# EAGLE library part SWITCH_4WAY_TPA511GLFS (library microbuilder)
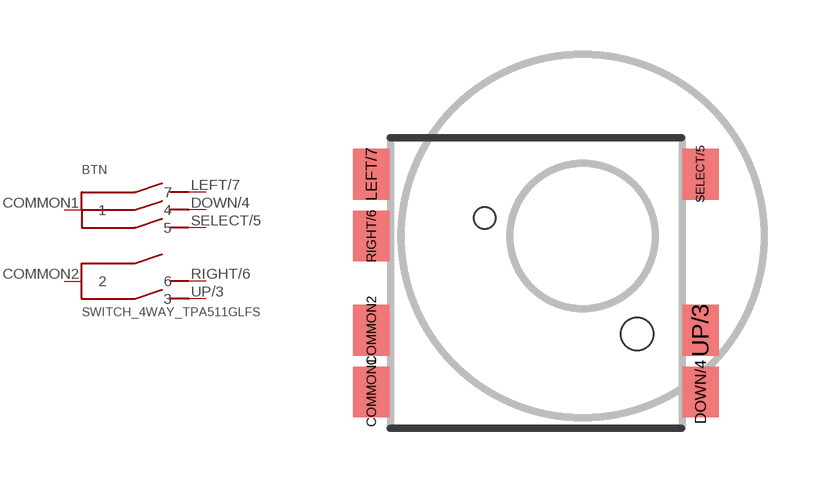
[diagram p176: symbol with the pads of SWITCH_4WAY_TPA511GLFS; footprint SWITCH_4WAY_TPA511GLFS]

Designator prefix BTN

## SWITCH_4WAY_TPA511GLFS  [SWITCH_4WAY_TPA511GLFS]
COMMON1  1
COMMON2  2
DOWN/4  4
LEFT/7  7
RIGHT/6  6
SELECT/5  5
UP/3  3

## Footprint SWITCH_4WAY_TPA511GLFS (pad centres in mm)
smd 1 x 1.4: COMMON1 -5.825,-4.3; COMMON2 -5.825,-2.6; DOWN/4 3.25,-4.3; LEFT/7 -5.825,1.7; RIGHT/6 -5.825,0; SELECT/5 3.25,1.7; UP/3 3.25,-2.6
hole 0.6 at -2.7,0.5
hole 0.9 at 1.5,-2.7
